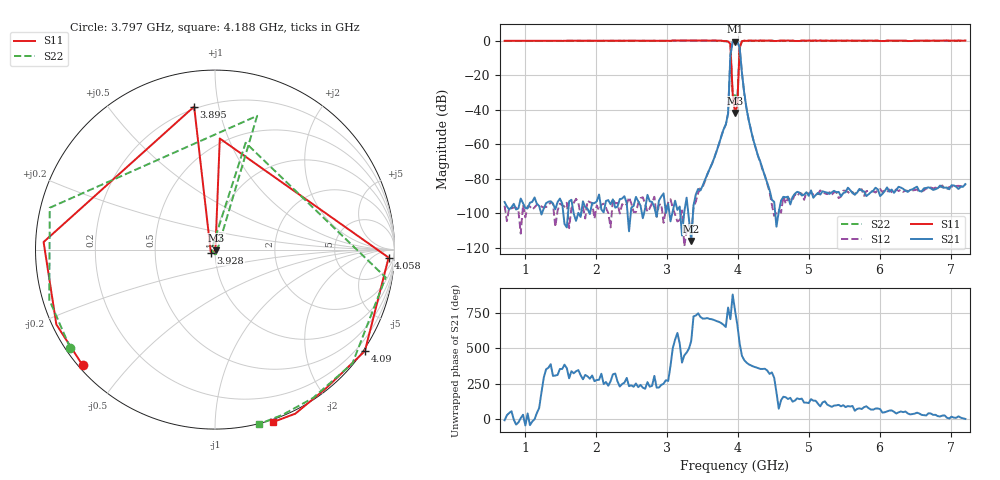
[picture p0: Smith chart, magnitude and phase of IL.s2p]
!Agilent Technologies,E8364B,MY43040703,A.07.50.48
!Agilent E8364B: A.07.50.48
!Date: Wednesday, April 10, 2024 13:06:41
!Correction: S11(Full 2 Port(1,2))
!S21(Full 2 Port(1,2))
!S12(Full 2 Port(1,2))
!S22(Full 2 Port(1,2))
!S2P File: Measurements: S11, S21, S12, S22:
# Hz S  dB  R 50
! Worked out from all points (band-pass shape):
!   201 points, 710 MHz to 7.21 GHz, reference 50 ohm
!   highest |S21| = -0.57 dB at 3.96 GHz (marker M1); lowest = -116.2 dB at 3.342 GHz (marker M2)
!   |S21| within 3 dB of the highest: 3.915 GHz to 4.024 GHz (108.3 MHz wide, 2.73 % of centre)
!   lowest |S11| = -42.0 dB at 3.96 GHz (marker M3), VSWR 1.02, Z = 50.7 - j0.46 ohm
!   |S11| at or under -10 dB: 3.904 GHz to 4.019 GHz (115.2 MHz wide, 2.91 % of centre)
!   |S22| runs from -34.0 to 0.1 dB; largest |S21 - S12| = 0.012
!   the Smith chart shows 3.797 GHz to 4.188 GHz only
!   S11 on the Smith chart (normalised r, x): 3.797 GHz: 0.01, -0.38; 3.895 GHz: 0.19, +0.85; 3.928 GHz: 0.95, -0.03; 4.058 GHz: 20, -29; 4.09 GHz: -0.05, -3.26; 4.188 GHz: -0.02, -1.39
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7.1e8  -0.05 121.9  -93.51 -10.5  -95.64 6.0  -0.12 119.2
1.2625e9  -0.01 78.8  -97.24 -68.3  -96.74 -12.4  -0.09 75.0
1.815e9  0.05 37.6  -93.10 -80.0  -96.25 -44.2  -0.03 33.0
2.3025e9  0.00 2.8  -96.21 -94.8  -94.03 -35.2  -0.00 -1.9
2.8875e9  0.02 -38.4  -92.65 -138.5  -95.21 -110.8  -0.06 -43.2
3.3425e9  0.14 -71.7  -116.16 -168.0  -111.98 -54.7  0.08 -77.0
3.5375e9  0.09 -90.7  -80.58 -9.5  -81.30 -1.2  0.08 -95.0
3.7e9  0.05 -112.4  -64.16 -27.4  -63.96 -26.4  0.08 -118.0
3.7975e9  -0.18 -138.9  -51.55 -53.5  -51.44 -53.2  -0.22 -145.8
3.8625e9  -0.39 177.5  -42.20 68.9  -42.13 69.1  -0.45 165.8
3.895e9  -1.88 98.3  -8.27 -14.2  -8.17 -13.9  -2.14 72.5
3.9275e9  -30.96 -144.6  -0.75 160.7  -0.64 160.5  -31.86 -76.6
3.96e9  -41.95 -34.6  -0.57 49.5  -0.47 49.6  -31.59 -91.6
3.9925e9  -37.59 -82.0  -0.59 -52.4  -0.52 -52.2  -33.98 -177.1
4.025e9  -4.16 87.5  -3.70 176.8  -3.58 176.7  -4.16 74.0
4.0575e9  -0.28 -2.6  -18.55 87.2  -18.40 87.4  -0.32 -9.3
4.09e9  0.07 -34.1  -30.20 55.9  -30.12 56.0  -0.05 -39.6
4.1875e9  0.12 -71.5  -52.23 17.9  -52.26 18.1  0.03 -76.0
4.415e9  0.09 -104.2  -82.41 -18.3  -83.06 -8.1  0.03 -108.0
5.065e9  0.08 -151.5  -91.05 128.5  -88.99 106.4  0.02 -154.9
6.1375e9  0.05 149.2  -87.57 58.2  -86.25 61.5  -0.01 143.8
7.21e9  0.13 93.2  -83.16 -1.1  -83.09 5.2  0.12 88.1
